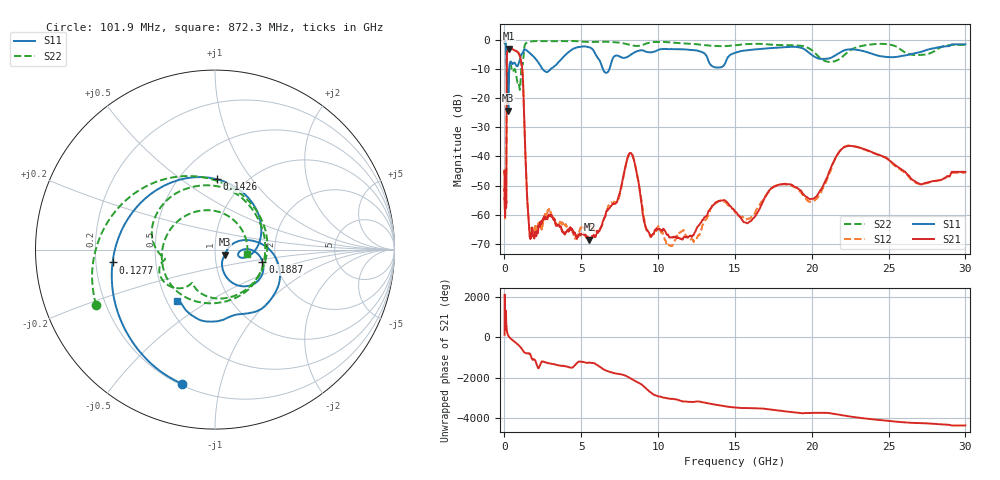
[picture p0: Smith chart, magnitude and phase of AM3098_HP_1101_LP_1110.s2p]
! Date/Time: Thu, Feb 28, 2019 8:46 AM
! Network Analyzer: Agilent Technologies E8364B Rev: A.07.50.67
! Sweep from 0.010 to 30.000 GHz, 1601 Points, Sweep Type: LOG
! Power Supply: 5.022 V, 0.002 A
# Hz S DB R 50
!freq MagS11 AngS11 MagS21 AngS21 MagS12 AngS12 MagS22 AngS22
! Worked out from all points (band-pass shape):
!   1601 points, 10 MHz to 30 GHz, reference 50 ohm
!   highest |S21| = -3.14 dB at 266.5 MHz (marker M1); lowest = -68.6 dB at 5.528 GHz (marker M2)
!   |S21| within 3 dB of the highest: 159.3 MHz to 1.028 GHz (868.7 MHz wide, 146 % of centre)
!   lowest |S11| = -24.3 dB at 252.2 MHz (marker M3), VSWR 1.13, Z = 55.6 - j3.12 ohm
!   |S11| at or under -10 dB: 148 MHz to 315.9 MHz (167.9 MHz wide, 72.4 % of centre); 2.474 GHz to 3.032 GHz (558.8 MHz wide, 20.3 % of centre); 6.394 GHz to 6.839 GHz (445.4 MHz wide, 6.73 % of centre)
!   |S22| runs from -17.2 to -0.5 dB; largest |S21 - S12| = 0.011
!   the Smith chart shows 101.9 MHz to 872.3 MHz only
!   S11 on the Smith chart (normalised r, x): 101.9 MHz: 0.21, -0.77; 127.7 MHz: 0.27, -0.06; 142.6 MHz: 0.75, +0.69; 188.7 MHz: 1.70, -0.25; 872.3 MHz: 0.56, -0.37
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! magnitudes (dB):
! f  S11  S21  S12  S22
! 10 MHz  -0.4  -45.5  -44.9  -0.6
! 38.04 MHz  -0.3  -57.9  -56.9  -0.9
! 101.9 MHz  -2.3  -55.0  -54.9  -2.7
! 127.7 MHz  -4.8  -42.4  -40.6  -6.2
! 142.6 MHz  -8.1  -16.8  -16.8  -10.8
! 144.7 MHz  -8.8  -14.3  -14.3  -10.9
! 188.7 MHz  -11.3  -4.0  -4.0  -10.0
! 252.2 MHz  -24.3  -3.2  -3.1  -11.0
! 266.5 MHz  -20.0  -3.1  -3.1  -10.8
! 550.5 MHz  -8.3  -3.4  -3.4  -10.9
! 872.3 MHz  -8.9  -4.3  -4.3  -14.8
! 1.178 GHz  -4.7  -11.3  -11.2  -8.7
! 1.63 GHz  -4.5  -66.5  -64.9  -0.7
! 2.084 GHz  -6.9  -66.6  -65.2  -0.5
! 5.528 GHz  -2.7  -68.6  -63.9  -0.8
! 7.926 GHz  -6.1  -42.3  -42.3  -1.5
! 8.416 GHz  -4.5  -41.1  -40.9  -2.1
! 9.349 GHz  -4.3  -65.7  -65.6  -1.2
! 10.76 GHz  -3.3  -67.8  -70.4  -1.0
! 20.1 GHz  -5.6  -54.5  -55.3  -4.1
! 22.56 GHz  -3.4  -36.4  -36.3  -3.5
! 30 GHz  -1.6  -45.3  -45.6  -1.8
